(* Logix 5000 AddOnInstructionDefinition export Banner_IOLM_TL50; software revision 32.00 *)

TYPE Banner_TL50_MSG_Data :   // UDT used with the AOI that changes the TL50 IO-Link unit between operating modes.
STRUCT
   Source : SINT[15];
   Destination : SINT[15];
   Change : BOOL;
END_STRUCT
END_TYPE

ADD_ON_INSTRUCTION Banner_IOLM_TL50   (* revision 1.0, vendor Banner Engineering *)
// AOI that controls an IO-Link master to change the TL50 Pro's Operation Mode.
VAR_IN_OUT
   MSG : MESSAGE; {required}   // Message used to send parameter updates to a device plugged into an Allen Bradley IO-Link Master.
   MSG_Data : Banner_TL50_MSG_Data; {required}
END_VAR
VAR_INPUT
   Port : DINT;
   Mode : DINT;
   IOL_Master : DINT;
END_VAR
VAR_OUTPUT
   Pass : BOOL; {access Read Only}
   Fail : BOOL;
   Error : BOOL;
END_VAR
VAR
   Lock : DINT; {access None}
   Current_Port : INT; {access None}   // Current port to communicate with via the IO-Link Master.
   Message_Timer : TIMER := (PRE := 100); {access None}
   Message_Timer2 : TIMER := (PRE := 5000); {access None}
END_VAR

ROUTINE Logic   (* ladder *)
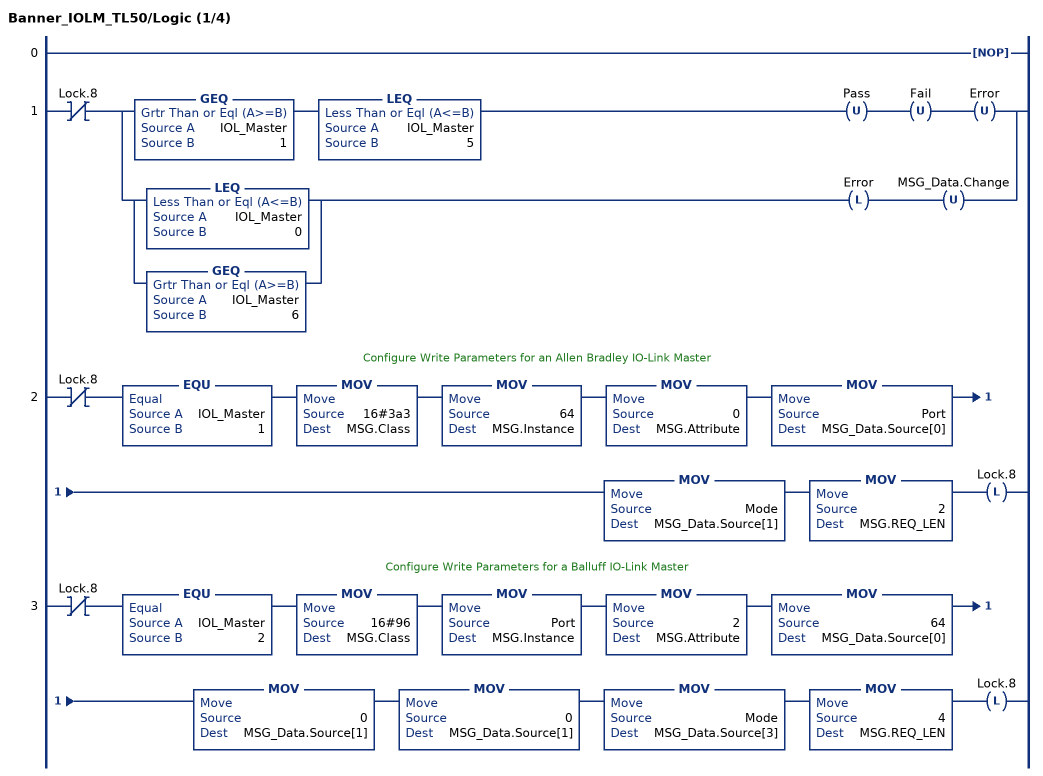
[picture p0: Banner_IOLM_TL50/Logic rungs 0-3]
   0: NOP();
   1: XIO(Lock.8)[GEQ(IOL_Master,1) LEQ(IOL_Master,5) OTU(Pass) OTU(Fail) OTU(Error) ,[LEQ(IOL_Master,0) ,GEQ(IOL_Master,6) ] OTL(Error) OTU(MSG_Data.Change) ];
   // Configure Write Parameters for an Allen Bradley IO-Link Master
   2: XIO(Lock.8)EQU(IOL_Master,1)MOV(16#3a3,MSG.Class)MOV(64,MSG.Instance)MOV(0,MSG.Attribute)MOV(Port,MSG_Data.Source[0])MOV(Mode,MSG_Data.Source[1])MOV(2,MSG.REQ_LEN)OTL(Lock.8);
   // Configure Write Parameters for a Balluff IO-Link Master
   3: XIO(Lock.8)EQU(IOL_Master,2)MOV(16#96,MSG.Class)MOV(Port,MSG.Instance)MOV(2,MSG.Attribute)MOV(64,MSG_Data.Source[0])MOV(0,MSG_Data.Source[1])MOV(0,MSG_Data.Source[1])MOV(Mode,MSG_Data.Source[3])MOV(4,MSG.REQ_LEN)OTL(Lock.8);
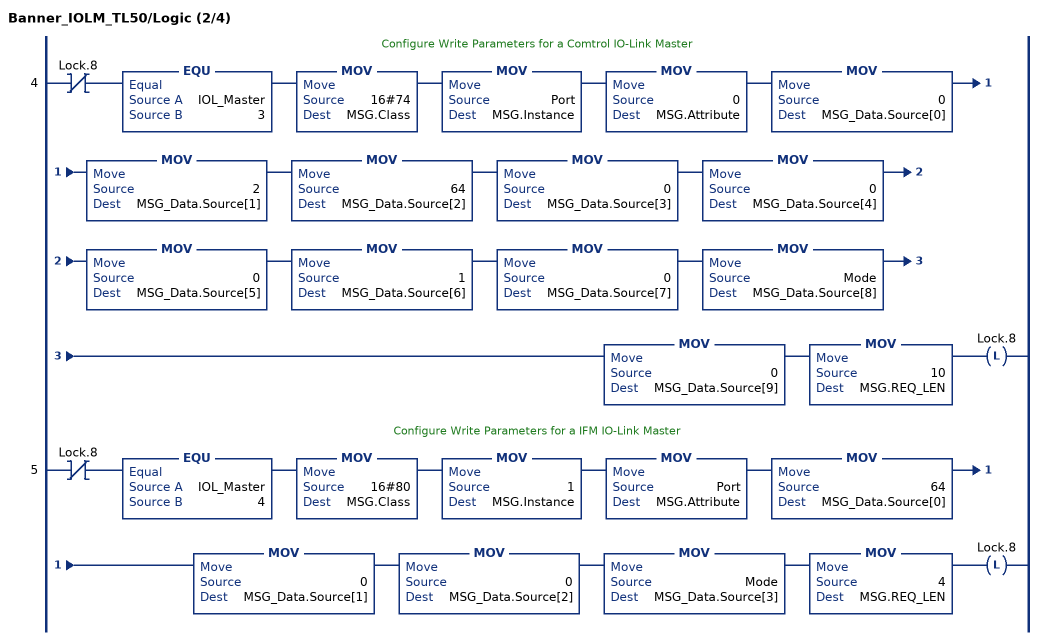
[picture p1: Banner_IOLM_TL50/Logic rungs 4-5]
   // Configure Write Parameters for a Comtrol IO-Link Master
   4: XIO(Lock.8)EQU(IOL_Master,3)MOV(16#74,MSG.Class)MOV(Port,MSG.Instance)MOV(0,MSG.Attribute)MOV(0,MSG_Data.Source[0])MOV(2,MSG_Data.Source[1])MOV(64,MSG_Data.Source[2])MOV(0,MSG_Data.Source[3])MOV(0,MSG_Data.Source[4])MOV(0,MSG_Data.Source[5])MOV(1,MSG_Data.Source[6])MOV(0,MSG_Data.Source[7])MOV(Mode,MSG_Data.Source[8])MOV(0,MSG_Data.Source[9])MOV(10,MSG.REQ_LEN)OTL(Lock.8);
   // Configure Write Parameters for a IFM IO-Link Master
   5: XIO(Lock.8)EQU(IOL_Master,4)MOV(16#80,MSG.Class)MOV(1,MSG.Instance)MOV(Port,MSG.Attribute)MOV(64,MSG_Data.Source[0])MOV(0,MSG_Data.Source[1])MOV(0,MSG_Data.Source[2])MOV(Mode,MSG_Data.Source[3])MOV(4,MSG.REQ_LEN)OTL(Lock.8);
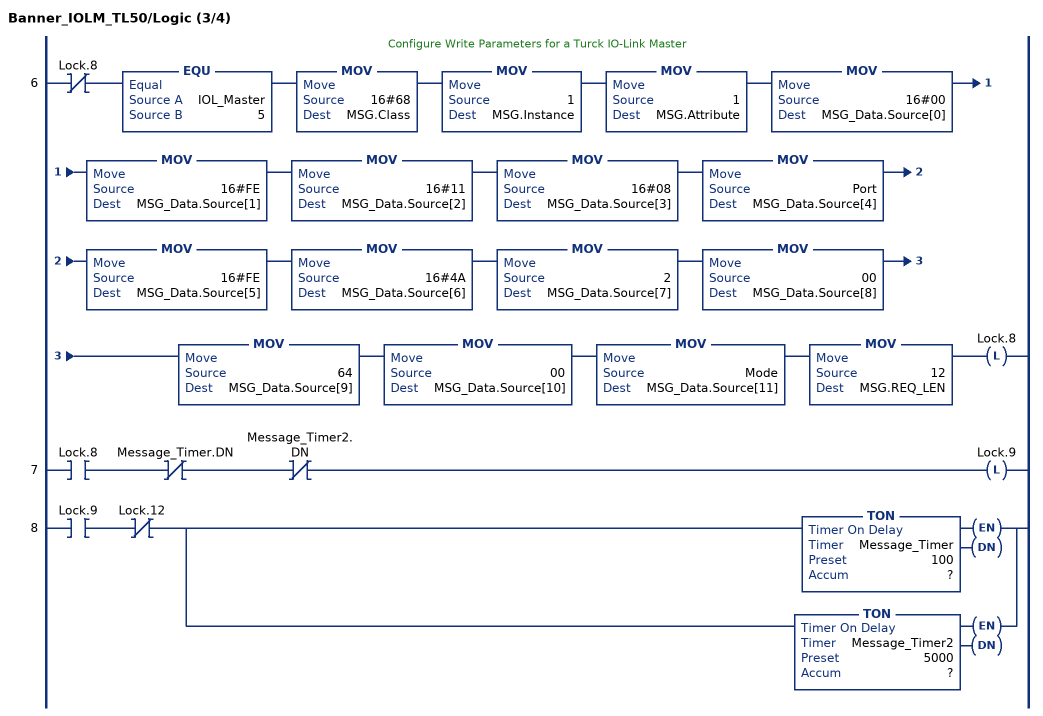
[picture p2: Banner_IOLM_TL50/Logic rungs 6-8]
   // Configure Write Parameters for a Turck IO-Link Master
   6: XIO(Lock.8)EQU(IOL_Master,5)MOV(16#68,MSG.Class)MOV(1,MSG.Instance)MOV(1,MSG.Attribute)MOV(16#00,MSG_Data.Source[0])MOV(16#FE,MSG_Data.Source[1])MOV(16#11,MSG_Data.Source[2])MOV(16#08,MSG_Data.Source[3])MOV(Port,MSG_Data.Source[4])MOV(16#FE,MSG_Data.Source[5])MOV(16#4A,MSG_Data.Source[6])MOV(2,MSG_Data.Source[7])MOV(00,MSG_Data.Source[8])MOV(64,MSG_Data.Source[9])MOV(00,MSG_Data.Source[10])MOV(Mode,MSG_Data.Source[11])MOV(12,MSG.REQ_LEN)OTL(Lock.8);
   7: XIC(Lock.8)XIO(Message_Timer.DN)XIO(Message_Timer2.DN)OTL(Lock.9);
   8: XIC(Lock.9)XIO(Lock.12)[TON(Message_Timer,?,?) ,TON(Message_Timer2,?,?) ];
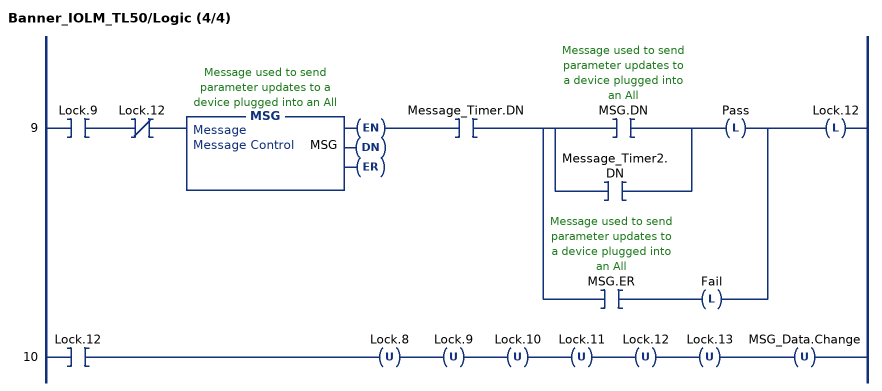
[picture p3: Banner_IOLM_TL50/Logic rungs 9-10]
   9: XIC(Lock.9)XIO(Lock.12)MSG(MSG)XIC(Message_Timer.DN)[[XIC(MSG.DN) ,XIC(Message_Timer2.DN) ] OTL(Pass) ,XIC(MSG.ER) OTL(Fail) ]OTL(Lock.12);
   10: XIC(Lock.12)OTU(Lock.8)OTU(Lock.9)OTU(Lock.10)OTU(Lock.11)OTU(Lock.12)OTU(Lock.13)OTU(MSG_Data.Change);
END_ROUTINE
END_ADD_ON_INSTRUCTION
